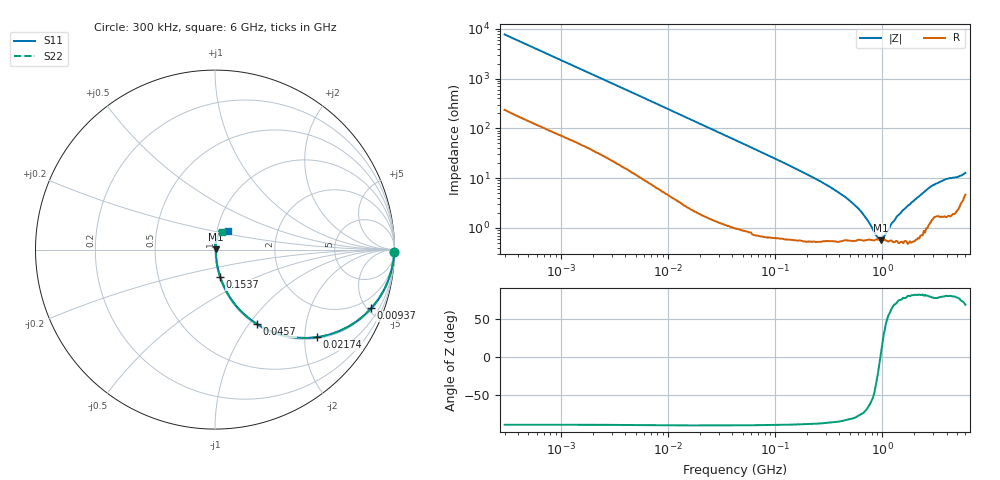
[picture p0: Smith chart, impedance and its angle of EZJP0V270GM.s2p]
!*** S-Parameter ***
!Copyright  (C)  Panasonic Corporation
!Multilaryer Varistors, Chip Type  Port assignments : Series-thru
!  1  o---GGG---o  2
!Parts No. : EZJP0V270GM  GND o---------o GND
# HZ S RI R 50
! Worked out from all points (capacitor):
!   401 points, 300 kHz to 6 GHz, reference 50 ohm
!   read as one part in series: C = 68.2 pF near 315.2 kHz
!   lowest |Z| = 565 mohm at 984.5 MHz (marker M1)
!   series resonance near 966.1 MHz, so ESL is about 400 pH
!   S11 on the Smith chart (normalised r, x): 300 kHz: open; 9.37 MHz: 1.10, -5.28; 21.74 MHz: 1.04, -2.29; 45.7 MHz: 1.02, -1.09; 153.7 MHz: 1.01, -0.31; 6 GHz: 1.14, +0.23
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300000  0.9994 -0.0136  0.000567 0.0129  0.000572 0.0129  0.9991 -0.0134
1575955  0.9935 -0.0649  0.00625 0.0651  0.00626 0.0651  0.9932 -0.0652
8278775  0.8944 -0.2979  0.1058 0.2976  0.1058 0.2977  0.8938 -0.2979
9369770  0.8701 -0.3273  0.1301 0.3269  0.1302 0.3271  0.8694 -0.3271
2.174284e7  0.5669 -0.4878  0.4328 0.4879  0.4332 0.4882  0.5663 -0.4878
4.348989e7  0.2511 -0.4253  0.7479 0.4255  0.7482 0.4258  0.2506 -0.4248
4.569764e7  0.2333 -0.4143  0.7655 0.4147  0.766 0.415  0.2328 -0.4139
7.685952e7  0.099 -0.2893  0.8998 0.289  0.9001 0.2892  0.0988 -0.289
1.537338e8  0.029 -0.1521  0.9695 0.1531  0.9699 0.1532  0.0289 -0.1519
2.228734e8  0.0151 -0.1021  0.9829 0.1036  0.9834 0.1038  0.015 -0.102
4.242534e8  0.0065 -0.0437  0.9916 0.0469  0.9917 0.0469  0.00666 -0.0436
5.853406e8  0.00507 -0.0231  0.9927 0.0269  0.993 0.0269  0.00553 -0.0229
7.497807e8  0.00436 -0.00994  0.9927 0.0139  0.9932 0.0137  0.00518 -0.00943
8.698622e8  0.00353 -0.00292  0.9925 0.00665  0.9927 0.00622  0.00481 -0.00227
9.369307e8  0.00344 0.000168  0.9925 0.00323  0.9927 0.00278  0.00492 0.000848
9.844927e8  0.00288 0.00217  0.9924 0.00116  0.9926 0.00064  0.00436 0.00284
1.170796e9  0.00242 0.00886  0.9921 -0.00711  0.9925 -0.00757  0.00421 0.00971
1.463031e9  0.00117 0.0176  0.9917 -0.0181  0.9918 -0.0187  0.00357 0.0182
3.395014e9  0.0273 0.0947  0.9804 -0.061  0.9772 -0.0607  0.0217 0.0932
4.13868e9  0.0275 0.1081  0.9752 -0.0753  0.9726 -0.0724  0.0238 0.1119
5.171722e9  0.0253 0.0971  0.9572 -0.102  0.9589 -0.0997  0.0245 0.0951
6e9  0.0744 0.1014  0.9408 -0.1159  0.946 -0.1115  0.0403 0.0984
